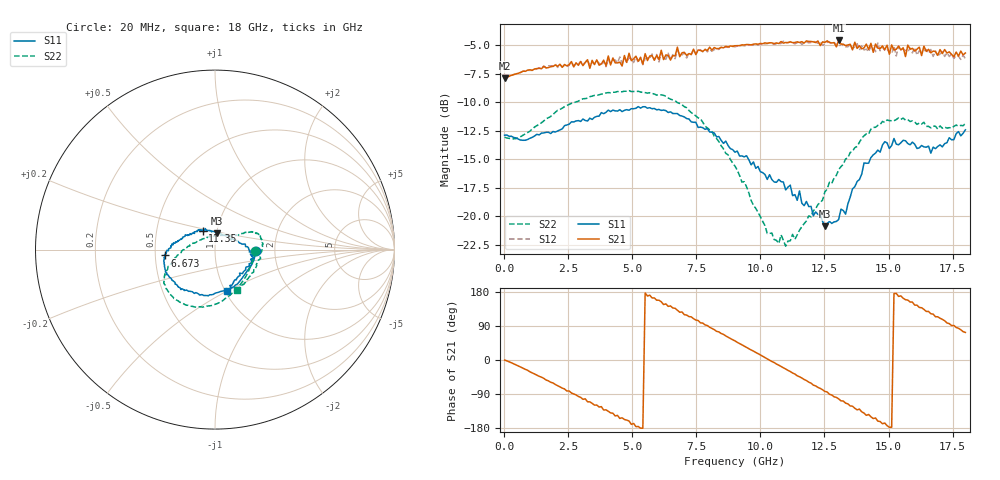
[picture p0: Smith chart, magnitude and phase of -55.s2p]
!Agilent Technologies,N5230A,US43500223,A.07.50.48
!Agilent N5230A: A.07.50.48
!Date: Monday, January 11, 2016 18:27:20
!Correction: S11(Full 2 Port(1,2))
!S21(Full 2 Port(1,2))
!S12(Full 2 Port(1,2))
!S22(Full 2 Port(1,2))
!S2P File: Measurements: S11, S21, S12, S22:
# Hz S  dB  R 50
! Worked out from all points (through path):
!   201 points, 20 MHz to 18 GHz, reference 50 ohm
!   highest |S21| = -4.56 dB at 13.06 GHz (marker M1); lowest = -7.9 dB at 20 MHz (marker M2)
!   group delay of S21, straight-line fit = 101 ps
!   lowest |S11| = -20.9 dB at 12.52 GHz (marker M3), VSWR 1.20, Z = 50 + j9.08 ohm
!   |S11| at or under -10 dB: start of sweep to end of sweep
!   |S22| runs from -22.6 to -9.0 dB; largest |S21 - S12| = 0.089
!   S11 on the Smith chart (normalised r, x): 20 MHz: 1.59, -0.02; 6.673 GHz: 0.56, -0.04; 11.35 GHz: 0.85, +0.18; 18 GHz: 1.02, -0.50
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2e7  -12.88 -1.7  -7.88 -0.2  -7.88 -0.3  -13.05 -1.9
1.5483e9  -12.68 -64.9  -6.84 -48.4  -6.79 -49.0  -11.62 -69.4
2.6271e9  -11.70 -98.2  -6.41 -87.1  -6.45 -87.1  -10.08 -94.1
3.0766e9  -11.46 -108.9  -6.77 -103.7  -6.66 -103.8  -9.68 -102.2
4.0655e9  -10.67 -130.4  -5.92 -135.3  -6.25 -135.7  -9.14 -118.6
4.515e9  -10.64 -139.0  -6.46 -154.2  -6.01 -154.2  -9.08 -125.3
5.5039e9  -10.38 -155.7  -5.72 176.9  -6.16 176.0  -9.14 -139.2
6.0433e9  -10.62 -164.4  -6.23 157.7  -6.45 153.5  -9.33 -145.7
6.6726e9  -10.97 -173.4  -5.92 136.4  -6.16 132.6  -9.85 -151.4
7.8413e9  -12.36 172.9  -5.36 92.7  -5.31 89.6  -12.08 -163.2
9.01e9  -14.37 160.7  -5.02 50.4  -5.12 47.1  -15.59 178.0
1.02686e10  -16.76 141.6  -4.81 2.9  -4.84 -0.7  -21.51 132.5
1.13474e10  -18.09 123.6  -4.74 -37.1  -4.86 -42.2  -22.02 74.8
1.20666e10  -19.95 100.4  -4.68 -66.3  -4.63 -68.9  -19.49 47.8
1.25161e10  -20.87 84.6  -4.73 -82.8  -4.88 -86.1  -17.86 37.2
1.30555e10  -20.27 52.2  -4.56 -102.7  -5.13 -108.0  -15.91 32.3
1.41343e10  -15.34 5.8  -4.88 -146.0  -5.32 -147.5  -12.77 25.3
1.45838e10  -14.18 -1.5  -5.24 -161.3  -4.78 -164.6  -12.01 21.0
1.50333e10  -14.04 -7.1  -5.77 -177.5  -5.60 177.4  -11.60 16.6
1.57525e10  -13.61 -22.4  -4.97 158.1  -5.56 152.8  -11.51 4.1
1.66515e10  -14.45 -43.8  -5.65 122.1  -5.35 115.7  -12.24 -19.8
1.8e10  -12.40 -73.4  -5.66 72.8  -6.17 65.5  -11.84 -61.3
